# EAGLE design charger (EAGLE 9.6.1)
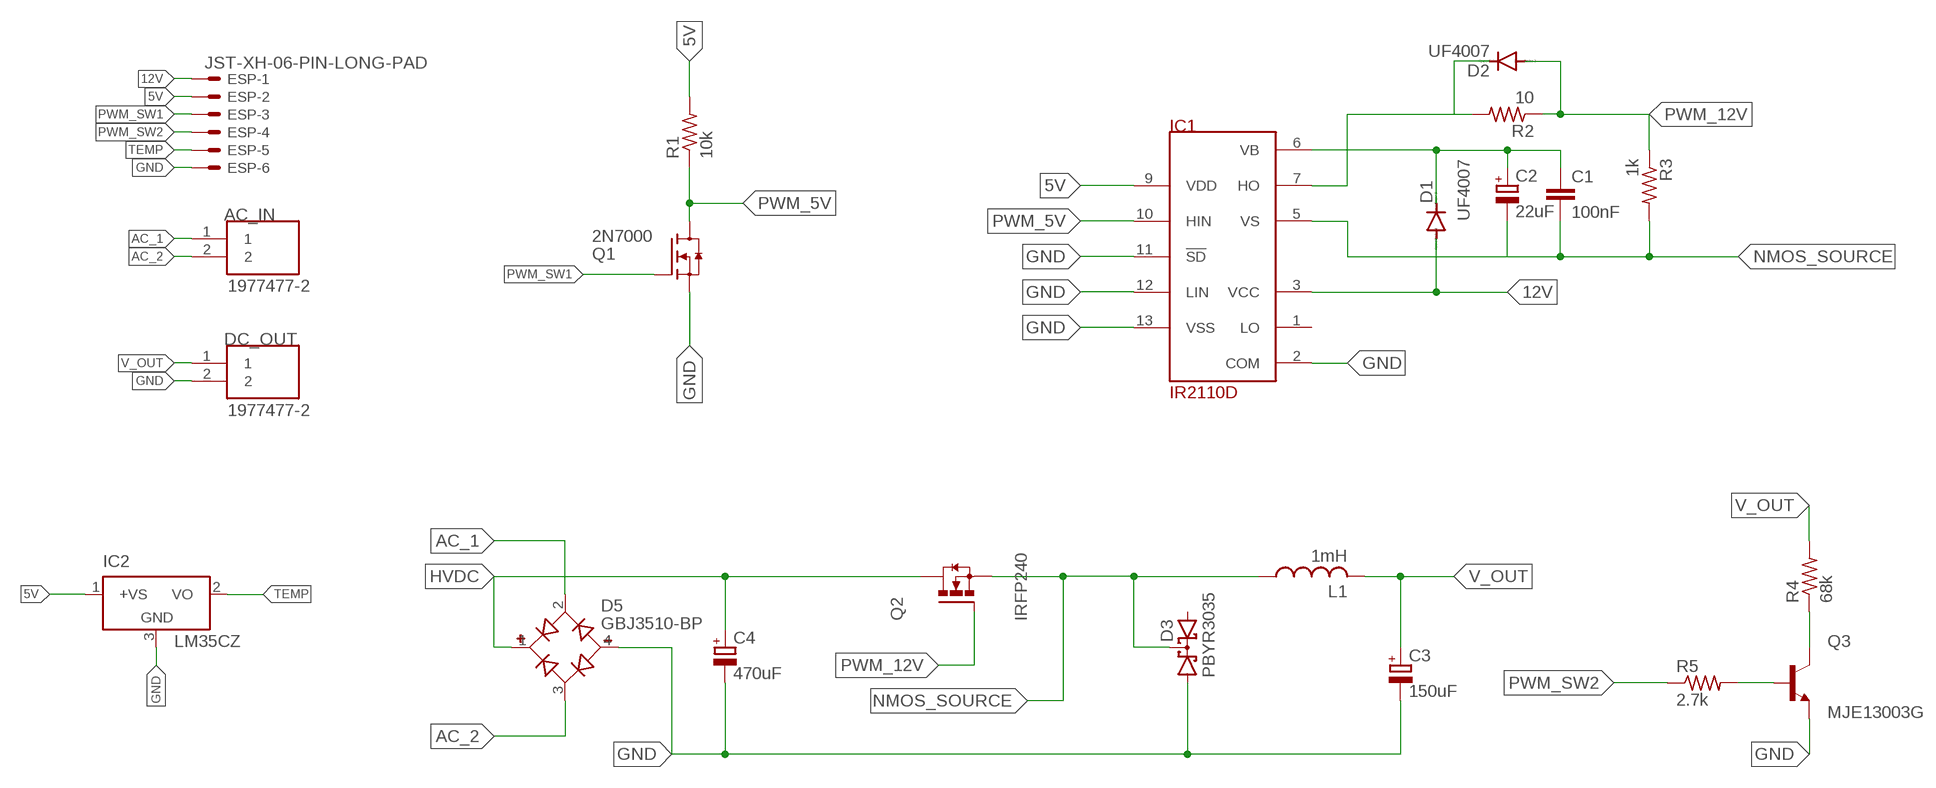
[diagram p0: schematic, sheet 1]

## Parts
AC_IN  1977477-2  [TE_1977477-2]
C1  100nF  C-EU025-025X050  [C025-025X050]
C2  22uF  CPOL-EUE2,5-6E  [E2,5-6E]
C3  150uF  CPOL-EUE7.5-18  [E7,5-18]
C4  470uF  CPOL-EUE10-35  [EB35D]
D1  UF4007  BAS15  [DO34-7]
D2  UF4007  BAS15  [DO34-7]
D3  PBYR3035  [SOT93S]
D5  GBJ3510-BP  [DIOB_GBJ3510-BP]
DC_OUT  1977477-2  [TE_1977477-2]
ESP  JST-XH-06-PIN-LONG-PAD  [JST-XH-06-PACKAGE-LONG-PAD]
IC1  IR2110D  [DIL14]
IC2  LM35CZ  [TO92]
L1  1mH  L-USTJ7-U1  [TJ7-U1]
Q1  2N7000  [TO92]
Q2  IRFP240  [TO247AC]
Q3  MJE13003G  [TO229P780X300X1364-3]
R1  10k  R-US_0204/7  [0204/7]
R2  10  R-US_0204/7  [0204/7]
R3  1k  R-US_0204/7  [0204/7]
R4  68k  R-US_0204/7  [0204/7]
R5  2.7k  R-US_0204/7  [0204/7]

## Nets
5V: ESP.2 IC1.9(VDD) IC2.1(+VS) R1.2
12V: D1.A ESP.1 IC1.3(VCC)
AC_1: AC_IN.1 D5.2(AC1)
AC_2: AC_IN.2 D5.3(AC2)
GND: C3.- C4.- D3.A1 D5.4(-) DC_OUT.2 ESP.6 IC1.2(COM) IC1.11(!SD) IC1.12(LIN) IC1.13(VSS) IC2.3(GND) Q1.1(S) Q3.3(E)
HVDC: C4.+ D5.1(+) Q2.2(D)
N$2: D2.C IC1.7(HO) R2.2
N$3: Q3.2(C) R4.1
N$5: Q3.1(B) R5.2
NMOS_SOURCE: C1.2 C2.- D3.C IC1.5(VS) L1.1 Q2.3(S) R3.2
PWM_5V: IC1.10(HIN) Q1.3(D) R1.1
PWM_12V: D2.A Q2.1(G) R2.1 R3.1
PWM_SW1: ESP.3 Q1.2(G)
PWM_SW2: ESP.4 R5.1
TEMP: ESP.5 IC2.2(VO)
V_OUT: C3.+ DC_OUT.1 L1.2 R4.2
VB: C1.1 C2.+ D1.C IC1.6(VB)
Unconnected: D3.A2 IC1.1(LO)

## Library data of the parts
AC_IN DC_OUT = terminal_block:1977477-2: Check availability; AVAILABILITY: In Stock; COMMENT: 1977477-2; DESCRIPTION: Conn Barrier Strip 2 POS 8.25mm Solder ST Thru-Hole 15A/Contact Carton; MF: TE Connectivity; MP: 1977477-2; PACKAGE: None; PRICE: None; PURCHASE-URL: https://pricing.snapeda.com/search/part/1977477-2/?ref=eda
C1 = rcl:C-EU: CAPACITOR, European symbol; SPICEPREFIX: C
C2-C4 = rcl:CPOL-EU: POLARIZED CAPACITOR, European symbol; SPICEPREFIX: C
D1 D2 = diode:BAS15: DIODE
D3 = diode:PBYR3035: Dual DIODE common cathode
D5 = GBJ3510-BP:GBJ3510-BP: Diode Rectifier Bridge Single 1KV 35A 4-Pin(4+Tab) Case GBJ Bulk/Tube Check availability; AVAILABILITY: In Stock; DESCRIPTION: Bridge Rectifier Single Phase Standard 1 kV Through Hole GBJ; MF: Micro Commercial; MP: GBJ3510-BP; PACKAGE: SIP-4 Micro Commercial Co; PRICE: None; PURCHASE-URL: https://pricing.snapeda.com/search/part/GBJ3510-BP/?ref=eda
ESP = Rembrandt Electronics - JST XH Connectors v1-0:JST-XH-06-PIN: JST XH Connector 2 Pin Wire to board connector. Pitch: 2,54 mm, (0.100") Number of pins: 6 Created by Rembrandt Electronics www.rembrandtelectronics.com
IC1 = irs:IR2110
IC2 = lm35:LM35: Single-Supply Centigrade Temperature Sensor Vout = (10mV/°C x Temp °C) +5mmmV Source: http://www.national.com/ds/LM/LM35.pdf
L1 = custom_inductor:L-US: INDUCTOR, American symbol; SPICEPREFIX: L
Q1 = 2N7000:2N7000: Check prices; AVAILABILITY: In Stock; DESCRIPTION: N-Channel 60V 350mA (Tc) 1W (Tc) Through Hole TO-92-3; MF: STMicroelectronics; MP: 2N7000; PACKAGE: E-PKG AXIAL-LEADED-2 ON Semiconductor; PRICE: None
Q2 = IRFP240(TO-247):IRFP240: MOSFET N-CH 200V 20A TO-247AC Check availability; AVAILABILITY: In Stock; DESCRIPTION: N-Channel 200 V 20A (Tc) 150W (Tc) Through Hole TO-247AC; MF: Vishay Siliconix; MP: IRFP240; PACKAGE: TO-247 Vishay Siliconix; PRICE: None
Q3 = MJE13003G:MJE13003G: Bipolar (BJT) Transistor NPN 400V 1.5A 10MHz 1.4W Through Hole TO-225AA Check availability; AVAILABILITY: Not in stock; DESCRIPTION: Bipolar (BJT) Transistor NPN 400 V 1.5 A 10MHz 1.4 W Through Hole TO-126; MF: ON Semiconductor; MP: MJE13003G; PACKAGE: TO-126 ON Semiconductor; PRICE: None
R1-R5 = rcl:R-US_: RESISTOR, American symbol; SPICEPREFIX: R

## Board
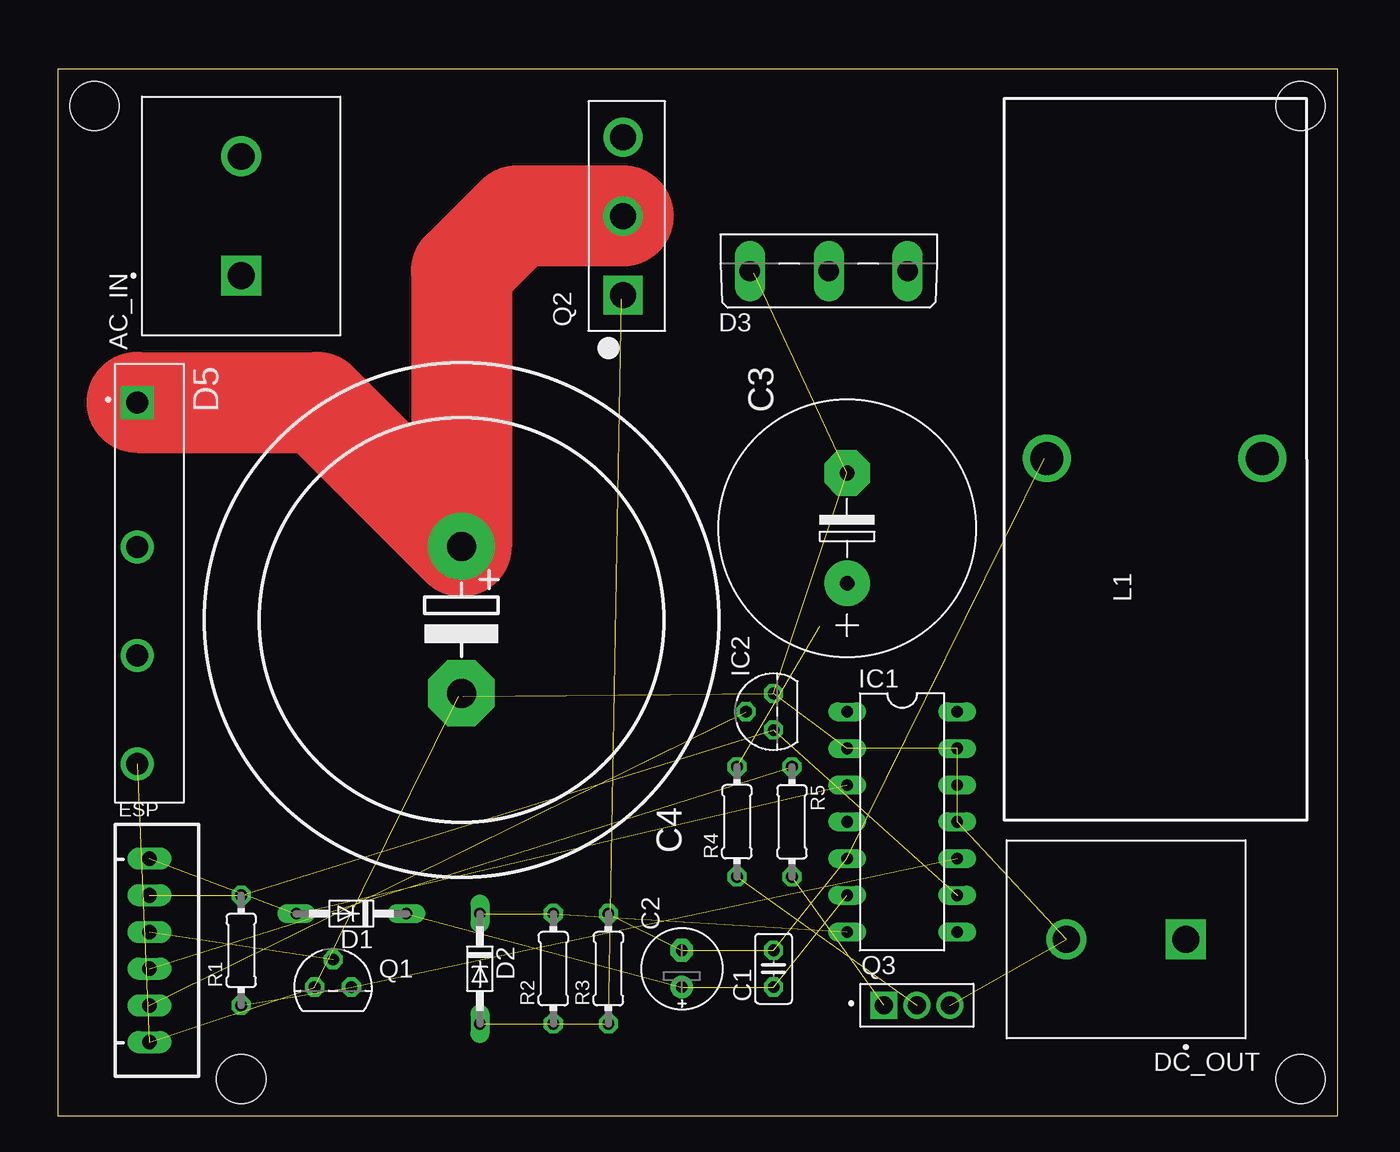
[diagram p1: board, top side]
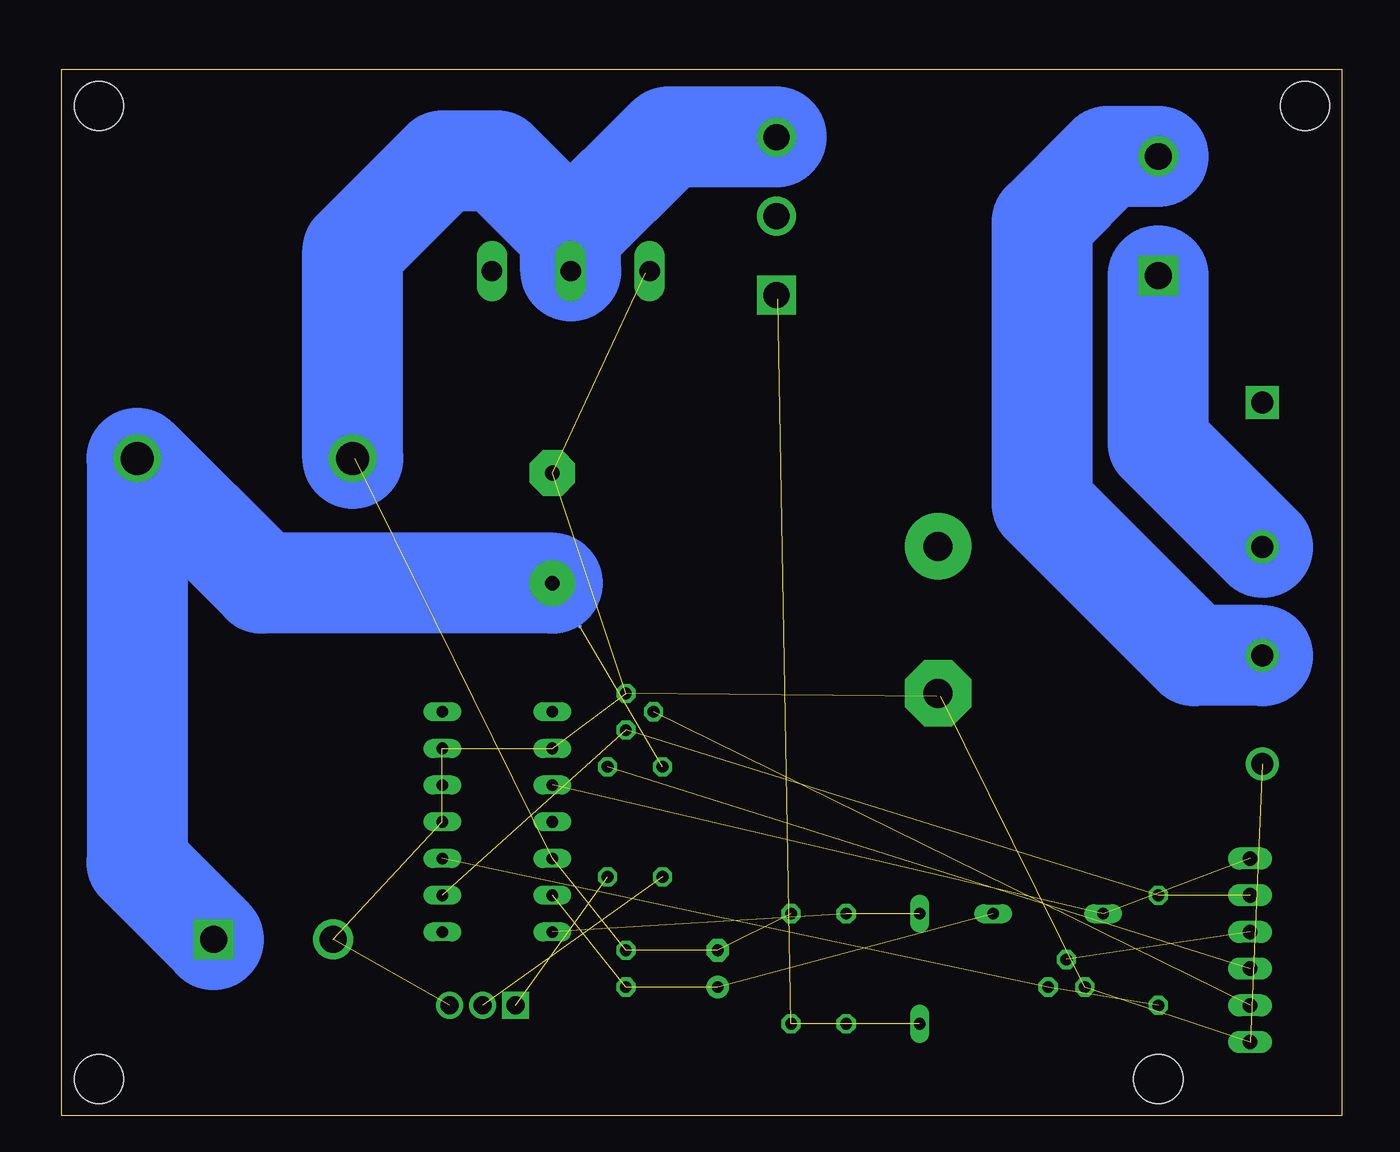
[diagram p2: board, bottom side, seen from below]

Size 88.57 x 72.38 mm. Coordinates in mm from the lower left corner, seen from the top.
Outline: 0,0 88.57,0 88.57,72.38 0,72.38 0,0
Copper layers (1*16): Top 0.035mm / dielectric 1.5mm / Bottom 0.035mm
Design rules "default *": minimum track width 12mil, minimum drill 0.35mm, track to track 12mil, track to pad 12mil, pad to pad 12mil, via to via 12mil, smd to smd 12mil, copper to edge 40mil, drill to drill 6mil, minimum pad ring 10mil, minimum via ring 8mil, stop-mask expansion 4mil, vias tented up to drill 0mil, thermal gap 10mil
Holes 3.4 mm at 2.54,69.85 85.98,69.85 12.7,2.54 85.98,2.54

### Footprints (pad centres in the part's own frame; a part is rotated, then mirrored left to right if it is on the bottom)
TE_1977477-2 = drill 1.85 square: 1 -4.13,0 | drill 1.85: 2 4.13,0
C025-025X050 = drill 0.813 octagon: 1 -1.27,0; 2 1.27,0
E2,5-6E = drill 0.813 pad 1.575: + -1.27,0 | drill 0.813 pad 1.575 octagon: - 1.27,0
E7,5-18 = drill 1.016 pad 3.15: + -3.81,0 | drill 1.016 pad 3.15 octagon: - 3.81,0
EB35D = drill 2.007 pad 4.597: + -5.08,0 | drill 2.007 pad 4.597 octagon: - 5.08,0
DO34-7 = drill 0.813 long: A 3.81,0; C -3.81,0
SOT93S = drill 1.397 long: A1 -5.461,-2.54; A2 5.461,-2.54; C 0,-2.54
DIOB_GBJ3510-BP = drill 1.51 pad 2.27 square: 1 -12.5,-0.85 | drill 1.51 pad 2.27: 2 -2.5,-0.85; 3 5,-0.85; 4 12.5,-0.85
JST-XH-06-PACKAGE-LONG-PAD = drill 1.016 long: 1 -6.35,0; 2 -3.81,0; 3 -1.27,0; 4 1.27,0; 5 3.81,0; 6 6.35,0
DIL14 = drill 0.813 long: 1 -7.62,-3.81; 2 -5.08,-3.81; 3 -2.54,-3.81; 4 0,-3.81; 5 2.54,-3.81; 6 5.08,-3.81; 7 7.62,-3.81; 8 7.62,3.81; 9 5.08,3.81; 10 2.54,3.81; 11 0,3.81; 12 -2.54,3.81; 13 -5.08,3.81; 14 -7.62,3.81
TO92 = drill 0.813 octagon: 1 -1.27,0; 2 0,1.905; 3 1.27,0
TJ7-U1 = drill 2.286: 1 -6.503,4.826; 2 8.408,4.826
TO247AC = drill 1.79 pad 2.69 square: 1 -5.46,0.255 | drill 1.79 pad 2.69: 2 0,0.255; 3 5.46,0.255
TO229P780X300X1364-3 = drill 1.25 square: 1 0,0 | drill 1.25: 2 2.29,0; 3 4.58,0
0204/7 = drill 0.813 octagon: 1 -3.81,0; 2 3.81,0

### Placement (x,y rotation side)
AC_IN  12.7,62.23 90 top
C1  49.53,10.16 90 top
C2  43.18,10.16 90 top
C3  54.61,40.64 90 top
C4  27.94,34.29 270 top
D1  20.32,13.97 180 top
D2  29.21,10.16 270 top
D3  53.34,60.96 0 top
D5  6.35,36.83 270 top
DC_OUT  73.91,12.19 180 top
ESP  6.35,11.43 270 top
IC1  58.42,20.32 270 top
IC2  49.53,27.94 90 top
L1  74.93,40.64 0 top
Q1  19.05,8.89 0 top
Q2  39.37,62.23 90 top
Q3  57.15,7.62 0 top
R1  12.7,11.43 90 top
R2  34.29,10.16 90 top
R3  38.1,10.16 90 top
R4  46.99,20.32 90 top
R5  50.8,20.32 270 top

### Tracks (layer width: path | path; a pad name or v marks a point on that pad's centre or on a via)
5V  (3 unrouted)
12V  (2 unrouted)
AC_1
  Bottom 6.985: D5.2 12.7,46.53 AC_IN.1
AC_2
  Bottom 6.985: D5.3 10.24,31.83 20.73,42.32 20.73,61.82 16.19,66.36 AC_IN.2
GND  (12 unrouted)
  Top 0.305: 27.74,29.01 C4.- 28.04,29.01 | 48.16,58.27 D3.A1
HVDC
  Top 6.985: Q2.2 31.75,62.23 27.94,58.42 C4.+ 17.98,49.33 D5.1
N$2  (2 unrouted)
N$3  (1 unrouted)
N$5  (1 unrouted)
NMOS_SOURCE  (4 unrouted)
  Top 0.305: 68.28,45.47 L1.1
  Bottom 6.985: Q2.3 46.61,67.69 53.34,60.96 | L1.1 68.43,59.84 62.23,66.04 58.42,66.04 53.34,60.96 | D3.C 53.34,60.96
PWM_5V  (2 unrouted)
PWM_12V  (3 unrouted)
  Bottom 0.305: 39.01,56.49 Q2.1
PWM_SW1  (1 unrouted)
PWM_SW2  (1 unrouted)
TEMP  (1 unrouted)
V_OUT  (1 unrouted)
  Bottom 0.305: 52.73,33.88 C3.+
  Bottom 6.985: DC_OUT.1 83.34,17.49 L1.2 74.7,36.83 C3.+
VB  (3 unrouted)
